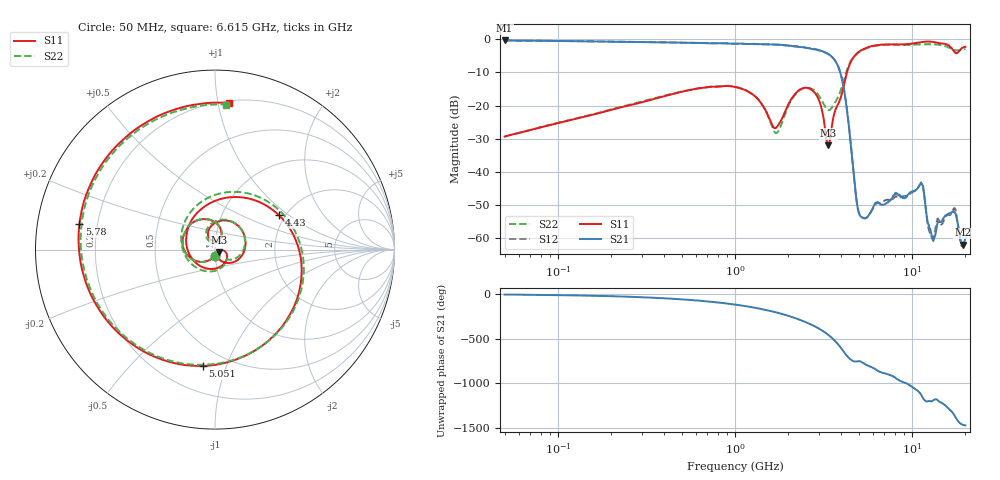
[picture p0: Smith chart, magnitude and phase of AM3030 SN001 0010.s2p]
# Hz S DB R 50
!freq MagS11 AngS11 MagS21 AngS21 MagS12 AngS12 MagS22 AngS22
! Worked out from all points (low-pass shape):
!   1601 points, 50 MHz to 20.05 GHz, reference 50 ohm
!   highest |S21| = -0.42 dB at 50 MHz (marker M1); lowest = -61.9 dB at 19.39 GHz (marker M2)
!   |S21| within 3 dB of the highest: start of sweep to 2.969 GHz
!   lowest |S11| = -32.0 dB at 3.37 GHz (marker M3), VSWR 1.05, Z = 52.1 - j1.46 ohm
!   |S11| at or under -10 dB: start of sweep to 4.3 GHz
!   |S22| runs from -29.3 to -1.5 dB; largest |S21 - S12| = 0.018
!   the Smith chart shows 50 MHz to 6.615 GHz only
!   S11 on the Smith chart (normalised r, x): 50 MHz: 1.00, -0.07; 4.43 GHz: 1.85, +0.85; 5.051 GHz: 0.37, -0.83; 5.78 GHz: 0.13, +0.09; 6.615 GHz: 0.22, +1.07
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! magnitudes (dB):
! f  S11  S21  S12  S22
! 50 MHz  -29.4  -0.4  -0.4  -29.3
! 135.9 MHz  -23.6  -0.6  -0.6  -23.5
! 369.6 MHz  -17.6  -1.0  -1.0  -17.5
! 1.005 GHz  -14.4  -1.4  -1.4  -14.4
! 1.351 GHz  -18.1  -1.5  -1.5  -18.1
! 1.711 GHz  -26.7  -1.6  -1.7  -28.3
! 2.182 GHz  -16.6  -2.1  -2.3  -16.8
! 2.722 GHz  -15.4  -3.0  -2.9  -15.0
! 3.023 GHz  -19.2  -3.5  -3.4  -17.5
! 3.37 GHz  -32.0  -4.5  -4.5  -21.4
! 3.959 GHz  -17.7  -10.5  -10.6  -15.5
! 4.43 GHz  -7.9  -27.5  -27.3  -7.5
! 4.829 GHz  -4.6  -47.1  -47.3  -4.7
! 5.051 GHz  -3.7  -52.7  -52.8  -3.9
! 5.78 GHz  -2.3  -52.5  -52.7  -2.4
! 6.615 GHz  -1.7  -49.6  -49.4  -1.8
! 7.402 GHz  -1.6  -48.8  -48.5  -1.7
! 11.26 GHz  -0.9  -43.4  -43.2  -1.6
! 12.84 GHz  -0.8  -58.3  -59.1  -1.5
! 17.32 GHz  -3.7  -51.8  -50.9  -3.3
! 19.39 GHz  -2.6  -61.9  -61.9  -3.1
! 20.05 GHz  -2.3  -59.9  -60.1  -3.0
